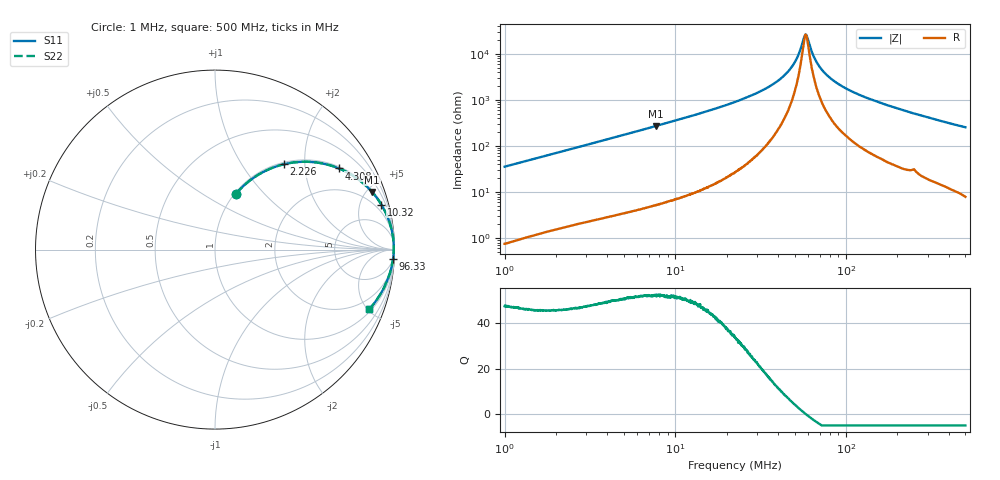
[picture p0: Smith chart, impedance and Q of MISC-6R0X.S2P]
!s-Parameter Generated by FASTRON Sdn. Bhd.
!FASTRON P/N : MISC-6R0X
!Keysight Technologies,E4991B,MY54100416,A.01.15
!Date: Mon Mar 16 10:32:36 2026
!Version  : Rev00 Mon Mar 16 10:32:36 2026
!Data & Calibration Information:
!PortZ  Port1:50+j0  Port2:50+j0
!When reading, reference impedance value at option line is always used.
!Remarks : This data is being provided solely for informational purposes.
!Freq	S11	S21	S12	S22
# Hz S dB R 50
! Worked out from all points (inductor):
!   1601 points, 1 MHz to 500 MHz, reference 50 ohm
!   read as one part in series: L = 5.64 uH near 1.032 MHz
!   highest Q = 52.4 at 7.654 MHz (marker M1), where L = 5.61 uH
!   self-resonance near 57.91 MHz
!   S11 on the Smith chart (normalised r, x): 1 MHz: 1.01, +0.71; 2.226 MHz: 1.03, +1.57; 4.308 MHz: 1.06, +3.02; 10.32 MHz: 1.14, +7.37; 96.33 MHz: 5, -38; 500 MHz: 1.16, -5.12
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1000000  -9.55 69.3  -0.58 -19.4  -0.58 -19.4  -9.55 69.3
1474639  -6.77 61.4  -1.12 -27.3  -1.12 -27.3  -6.77 61.4
2225832  -4.29 51.1  -2.17 -37.6  -2.17 -37.6  -4.29 51.1
2820919  -3.14 44.7  -3.06 -44.1  -3.06 -44.1  -3.14 44.7
4307824  -1.66 33.2  -5.24 -55.7  -5.24 -55.7  -1.66 33.2
7654427  -0.61 20.2  -9.24 -68.7  -9.24 -68.7  -0.61 20.2
7957584  -0.57 19.5  -9.54 -69.4  -9.54 -69.4  -0.57 19.5
1.032287e7  -0.35 15.1  -11.68 -73.8  -11.68 -73.8  -0.35 15.1
2.236068e7  -0.08 6.3  -19.23 -82.0  -19.23 -82.0  -0.08 6.3
3.323107e7  -0.04 3.3  -24.70 -83.5  -24.70 -83.5  -0.04 3.3
4.310858e7  -0.03 1.7  -30.45 -81.8  -30.45 -81.8  -0.03 1.7
5.035446e7  -0.03 0.8  -36.74 -75.2  -36.74 -75.2  -0.03 0.8
5.7687e7  -0.03 0.0  -48.38 -9.6  -48.38 -9.6  -0.03 0.0
5.950765e7  -0.03 -0.1  -46.93 31.6  -46.93 31.6  -0.03 -0.1
6.307767e7  -0.03 -0.5  -40.87 63.9  -40.87 63.9  -0.03 -0.5
6.764552e7  -0.04 -0.9  -36.15 73.7  -36.15 73.7  -0.04 -0.9
7.368004e7  -0.04 -1.4  -32.40 78.3  -32.40 78.3  -0.04 -1.4
8.278574e7  -0.05 -2.0  -28.93 80.6  -28.93 80.6  -0.05 -2.0
9.632587e7  -0.06 -3.0  -25.72 81.4  -25.72 81.4  -0.06 -3.0
1.244731e8  -0.08 -4.7  -21.79 81.2  -21.79 81.2  -0.08 -4.7
1.77937e8  -0.14 -7.5  -17.67 79.2  -17.67 79.2  -0.14 -7.5
5e8  -0.71 -21.1  -8.87 67.1  -8.87 67.1  -0.71 -21.1
